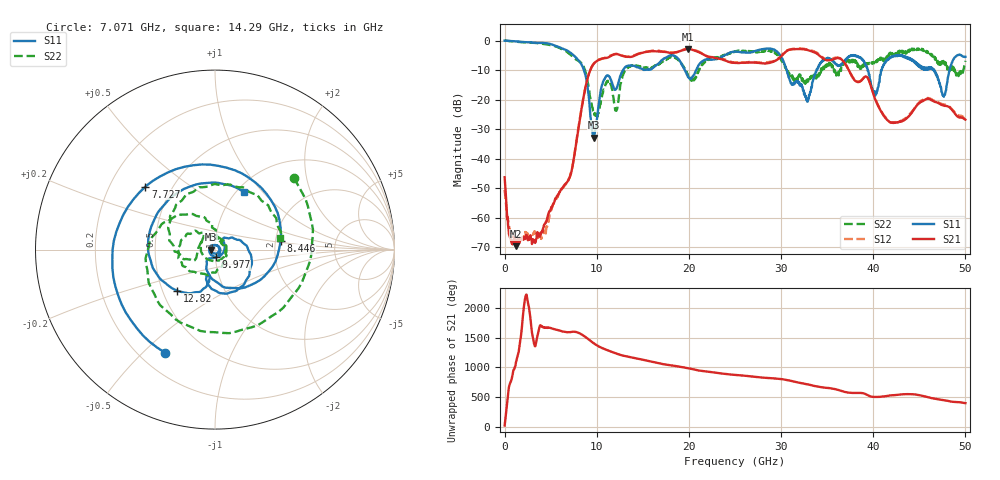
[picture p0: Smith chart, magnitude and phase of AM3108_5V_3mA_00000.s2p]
# Hz S DB R 50.0
!freq dBS11 angS11 dBS21 angS21 dBS12 angS12 dBS22 angS22
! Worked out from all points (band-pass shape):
!   1601 points, 10 MHz to 50 GHz, reference 50 ohm
!   highest |S21| = -2.82 dB at 19.94 GHz (marker M1); lowest = -69.6 dB at 1.197 GHz (marker M2)
!   |S21| within 3 dB of the highest: 11.11 GHz to 22.81 GHz (11.69 GHz wide, 68.9 % of centre); 29.84 GHz to 34.45 GHz (4.611 GHz wide, 14.3 % of centre)
!   lowest |S11| = -32.8 dB at 9.664 GHz (marker M3), VSWR 1.05, Z = 47.8 - j0.105 ohm
!   |S11| at or under -10 dB: 8.623 GHz to 12.85 GHz (4.223 GHz wide, 39.3 % of centre); 30.62 GHz to 33.85 GHz (3.227 GHz wide, 10 % of centre); 46.63 GHz to 48.29 GHz (1.658 GHz wide, 3.49 % of centre)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
!   |S22| runs from -26.1 to 0.1 dB; largest |S21 - S12| = 0.025
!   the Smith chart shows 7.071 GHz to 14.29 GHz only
!   S11 on the Smith chart (normalised r, x): 7.071 GHz: 0.30, -0.59; 7.727 GHz: 0.35, +0.34; 8.446 GHz: 2.14, +0.23; 9.977 GHz: 1.00, -0.09; 12.82 GHz: 0.60, -0.30; 14.29 GHz: 1.07, +0.80
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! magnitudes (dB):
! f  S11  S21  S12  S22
! 10 MHz  0.0  -46.2  -50.6  0.1
! 1.197 GHz  -0.2  -69.6  -68.4  -0.3
! 4.228 GHz  -0.8  -63.3  -64.2  -1.1
! 7.071 GHz  -3.9  -46.3  -46.2  -4.5
! 7.727 GHz  -5.6  -35.7  -35.5  -6.3
! 8.352 GHz  -8.1  -23.1  -23.0  -7.7
! 8.446 GHz  -8.7  -21.4  -21.3  -8.1
! 9.664 GHz  -32.8  -7.9  -7.9  -23.9
! 9.977 GHz  -27.4  -7.0  -6.8  -26.1
! 10.82 GHz  -13.1  -5.9  -5.9  -16.3
! 12.13 GHz  -16.3  -4.5  -4.5  -23.8
! 12.82 GHz  -10.2  -5.2  -5.1  -11.7
! 14.29 GHz  -8.9  -4.8  -4.7  -8.6
! 16.69 GHz  -7.8  -3.6  -3.4  -8.2
! 19.94 GHz  -12.3  -2.8  -2.7  -12.3
! 25 GHz  -3.6  -7.5  -7.4  -3.8
! 33.35 GHz  -15.5  -3.6  -3.4  -12.7
! 37.88 GHz  -4.9  -13.0  -12.9  -6.5
! 40.22 GHz  -18.6  -19.9  -19.6  -7.5
! 41.69 GHz  -6.1  -27.3  -27.3  -5.2
! 47.66 GHz  -19.0  -22.0  -21.7  -7.7
! 50 GHz  -5.5  -26.8  -26.9  -6.8
